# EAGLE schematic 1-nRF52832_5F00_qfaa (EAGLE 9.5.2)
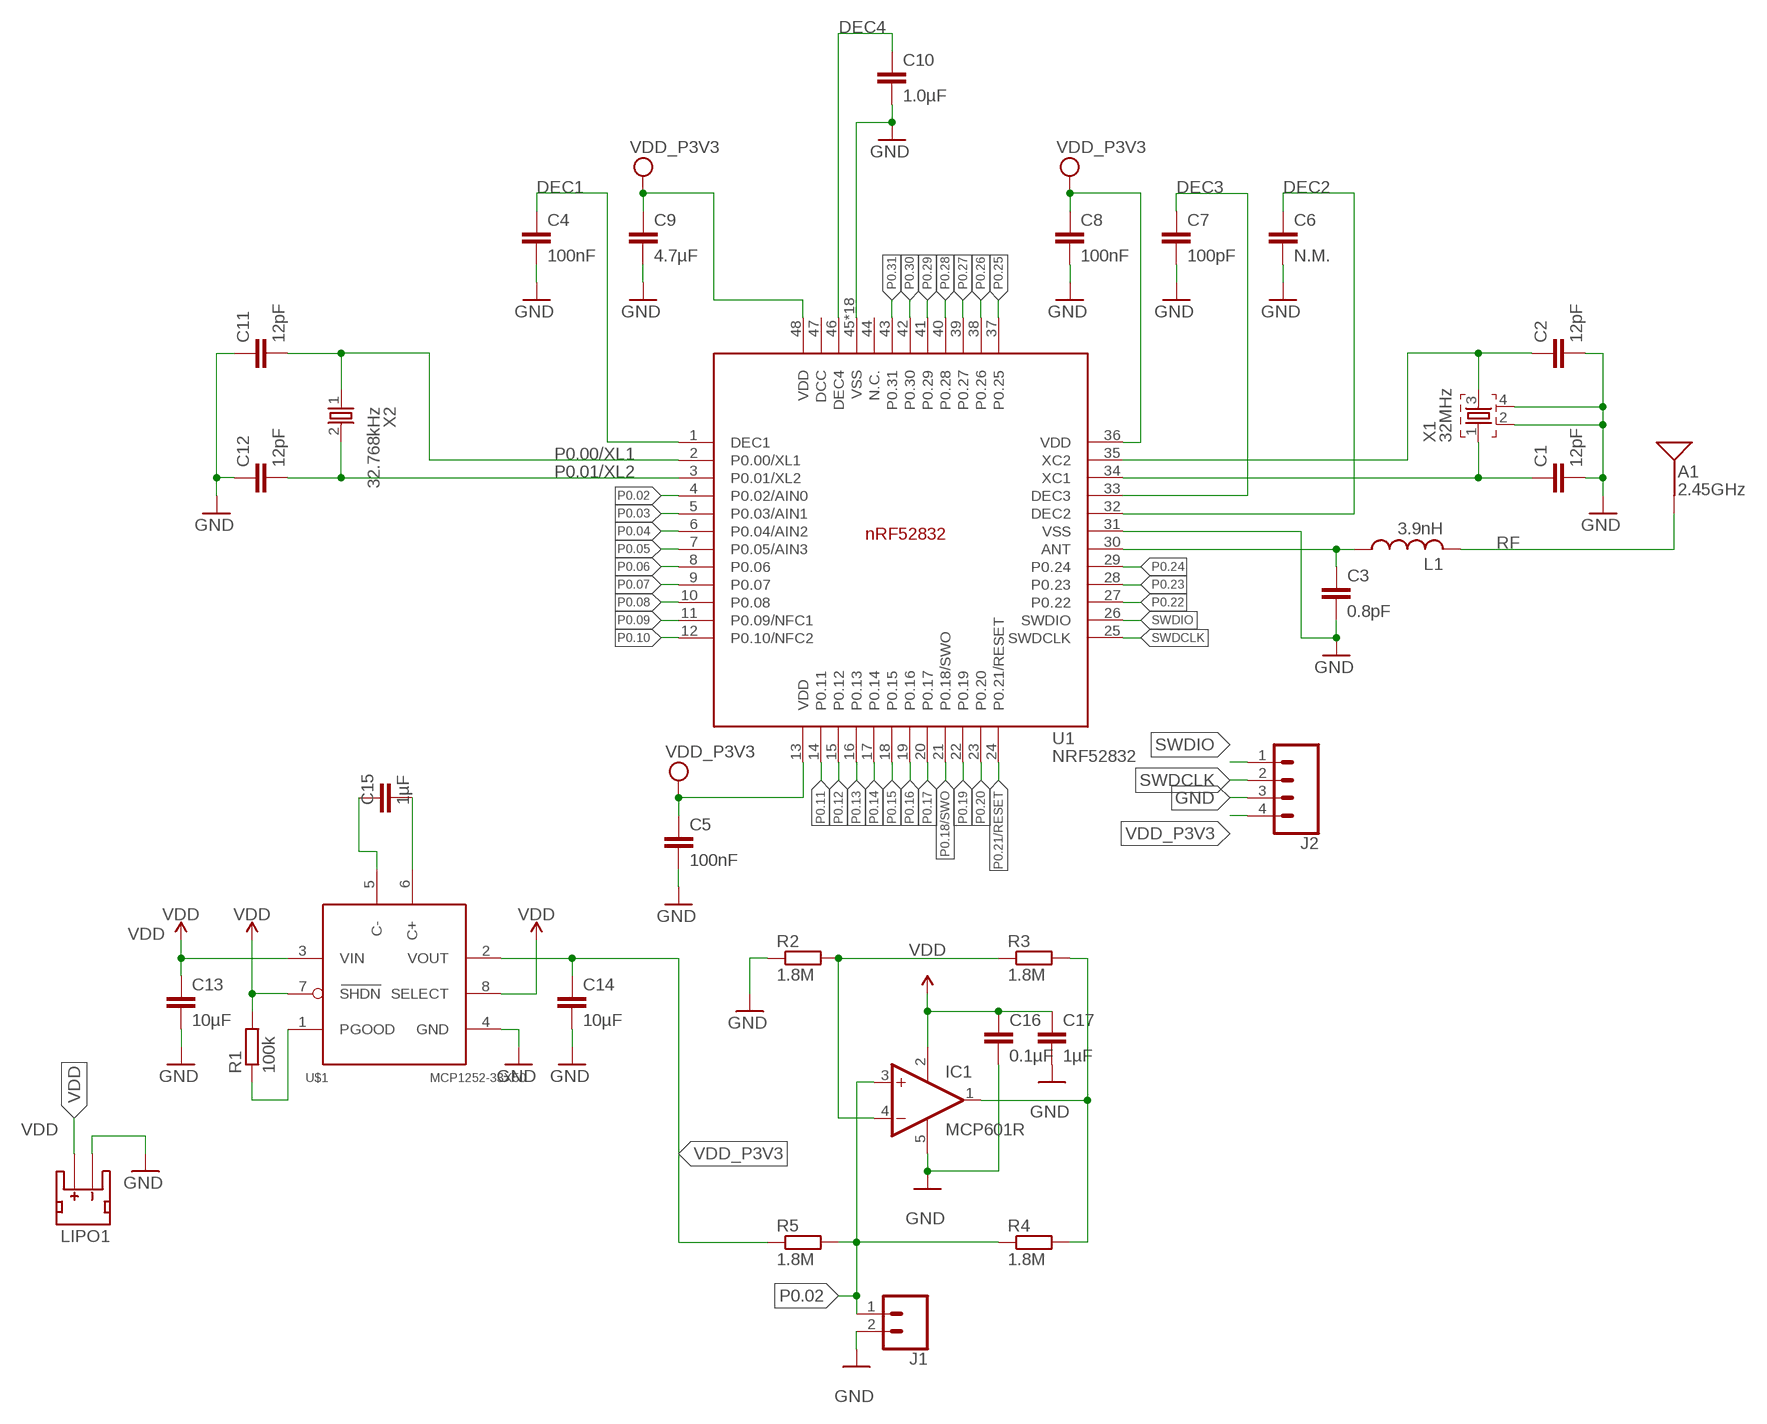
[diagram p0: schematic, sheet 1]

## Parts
A1  2.45GHz  ANTENNA2.4GHZ-6.5X2.2MM  [ANT-2.4GHZ-6.5X2.2MM]
C1  12pF  CAPACITOR_0402_N  [RESC0402_N]
C2  12pF  CAPACITOR_0402_N  [RESC0402_N]
C3  0.8pF  CAPACITOR_0402_N  [RESC0402_N]
C4  100nF  CAPACITOR_0402_N  [RESC0402_N]
C5  100nF  CAPACITOR_0402_N  [RESC0402_N]
C6  N.M.  CAPACITOR_0402_N  [RESC0402_N]
C7  100pF  CAPACITOR_0402_N  [RESC0402_N]
C8  100nF  CAPACITOR_0402_N  [RESC0402_N]
C9  4.7µF  CAPACITOR_0603_N  [RESC0603_N]
C10  1.0µF  CAPACITOR_0603_N  [RESC0603_N]
C11  12pF  CAPACITOR_0402_N  [RESC0402_N]
C12  12pF  CAPACITOR_0402_N  [RESC0402_N]
C13  10µF  C-EUC1206  [C1206]
C14  10µF  C-EUC1206  [C1206]
C15  1µF  C-EUC0805  [C0805]
C16  0.1µF  C-EUC0805  [C0805]
C17  1µF  C-EUC0805  [C0805]
IC1  MCP601R  [SOT23-5]
J1  CONN_02  [1X02]
J2  CONN_04  [1X04]
L1  3.9nH  INDUCTOR_0402_N  [RESC0402_N]
LIPO1  JST_2MM_MALE  [JST-2-SMD]
R1  100k  R-EU_R0805  [R0805]
R2  1.8M  R-EU_R0805  [R0805]
R3  1.8M  R-EU_R0805  [R0805]
R4  1.8M  R-EU_R0805  [R0805]
R5  1.8M  R-EU_R0805  [R0805]
U1  NRF52832  [QFN40P600X600X90-48_N]
U$1  MCP1252-33X50  [MSOP8]
X1  32MHz  XTAL_32MHZ  [BT-XTAL_2016_N]
X2  32.768kHz  XTAL_32KHZ  [XTAL_3215_N]

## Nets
ANT: C3.1 L1.1 U1.30(ANT)
C+: C15.2 U$1.6(C+)
C-: C15.1 U$1.5(C-)
DEC1: C4.1 U1.1(DEC1)
DEC2: C6.1 U1.32(DEC2)
DEC3: C7.1 U1.33(DEC3)
DEC4: C10.1 U1.46(DEC4)
GND: C1.2 C2.2 C3.2 C4.2 C5.2 C6.2 C7.2 C8.2 C9.2 C10.2 C11.1 C12.1 C13.2 C14.2 C16.2 C17.2 IC1.5(V-) J1.2 J2.3 LIPO1.1(-) R2.1 U1.31(VSS) U1.45(VSS) U1.PAD(VSS) U1.PAD@VIA01(VSS) U1.PAD@VIA02(VSS) U1.PAD@VIA03(VSS) U1.PAD@VIA04(VSS) U1.PAD@VIA05(VSS) U1.PAD@VIA06(VSS) U1.PAD@VIA07(VSS) U1.PAD@VIA08(VSS) U1.PAD@VIA09(VSS) U1.PAD@VIA10(VSS) U1.PAD@VIA11(VSS) U1.PAD@VIA12(VSS) U1.PAD@VIA13(VSS) U1.PAD@VIA14(VSS) U1.PAD@VIA15(VSS) U1.PAD@VIA16(VSS) U$1.4(GND) X1.2 X1.4
N$1: IC1.1(OUT) R3.2 R4.2
N$3: C2.1 U1.35(XC2) X1.3
N$4: R1.1 U$1.1(PGOOD)
N$6: IC1.4(-IN) R2.2 R3.1
P0.00/XL1: C11.2 U1.2(P0.00/XL1) X2.1
P0.01/XL2: C12.2 U1.3(P0.01/XL2) X2.2
P0.02: IC1.3(+IN) J1.1 R4.1 R5.2 U1.4(P0.02/AIN0)
P0.03: U1.5(P0.03/AIN1)
P0.04: U1.6(P0.04/AIN2)
P0.05: U1.7(P0.05/AIN3)
P0.06: U1.8(P0.06)
P0.07: U1.9(P0.07)
P0.08: U1.10(P0.08)
P0.09: U1.11(P0.09/NFC1)
P0.10: U1.12(P0.10/NFC2)
P0.11: U1.14(P0.11)
P0.12: U1.15(P0.12)
P0.13: U1.16(P0.13)
P0.14: U1.17(P0.14)
P0.15: U1.18(P0.15)
P0.16: U1.19(P0.16)
P0.17: U1.20(P0.17)
P0.18/SWO: U1.21(P0.18/SWO)
P0.19: U1.22(P0.19)
P0.20: U1.23(P0.20)
P0.21/RESET: U1.24(P0.21/RESET)
P0.22: U1.27(P0.22)
P0.23: U1.28(P0.23)
P0.24: U1.29(P0.24)
P0.25: U1.37(P0.25)
P0.26: U1.38(P0.26)
P0.27: U1.39(P0.27)
P0.28: U1.40(P0.28)
P0.29: U1.41(P0.29)
P0.30: U1.42(P0.30)
P0.31: U1.43(P0.31)
RF: A1.FEED(SIGNAL) L1.2
SWDCLK: J2.2 U1.25(SWDCLK)
SWDIO: J2.1 U1.26(SWDIO)
VDD: C13.1 C16.1 C17.1 IC1.2(V+) LIPO1.2(+) R1.2 U$1.3(VIN) U$1.7(SHDN) U$1.8(SELECT)
VDD_P3V3: C5.1 C8.1 C9.1 C14.1 J2.4 R5.1 U1.13(VDD) U1.36(VDD) U1.48(VDD) U$1.2(VOUT)
X1: C1.1 U1.34(XC1) X1.1
Unconnected: LIPO1.NC1(PAD1) LIPO1.NC2(PAD2) U1.44(N.C.) U1.47(DCC)

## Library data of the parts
A1 = SparkFun-RF:ANTENNA: Single-ended Antennae; PROD_ID: ANT-08187; SF_ID: WRL-00144
C1-C12 = Nordic_nRF:CAPACITOR: Generic chip capacitor
C13-C17 = rcl:C-EU: CAPACITOR, European symbol; SPICEPREFIX: C
IC1 = linear:MCP601: Single Op Amp 2.7V to 6.0V Single Supply CMOS Source: http://ww1.microchip.com/downloads/en/DeviceDoc/21314g.pdf
J1 = CalvEngIO-Connectors:CONN_02: Multi connection point. Often used as Generic Header-pin footprint for 0.1 inch spaced/style header connections
J2 = CalvEngIO-Connectors:CONN_04: Multi connection point. Often used as Generic Header-pin footprint for 0.1 inch spaced/style header connections On any of the 0.1 inch spaced packages, you can populate with these: Break Away Headers - Straight (PRT-00116) Break Away Male Headers - Right Angle (PRT-00553) Female Headers (PRT-00115)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; PROD_ID: CONN-09696
L1 = Nordic_nRF:INDUCTOR: Generic chip inductor
LIPO1 = CalvEngIO-Connectors:JST_2MM_MALE: JST 2MM MALE RA CONNECTOR Two pin, compact surface mount connector. Commonly used as a battery input connection point. We really like the solid locking feeling and high current rating on these small connectors. We use these all the time as battery connectors. Mates to single-cell LiPo batteries.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; PROD_ID: CONN-11443; SF_ID: PRT-08612
R1-R5 = rcl:R-EU_: RESISTOR, European symbol; SPICEPREFIX: R
U1 = Nordic_nRF:NRF52832: nRF52832 Features Single chip, highly flexible, 2.4 GHz multi-protocol SoC 32-bit ARM Cortex-M4F Processor 1.7v to 3.6v operation 512kB flash + 64kB RAM Supports concurrent Bluetooth Smart/ANT protocol operation On-chip NFC tag for Out-of-Band (OOB) pairing Up to +4dBm output power -96dBm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
U$1 = microchip-mcp125x-xxx:MCP1252-33X50
X1 = Nordic_nRF:XTAL_32MHZ
X2 = Nordic_nRF:XTAL_32KHZ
